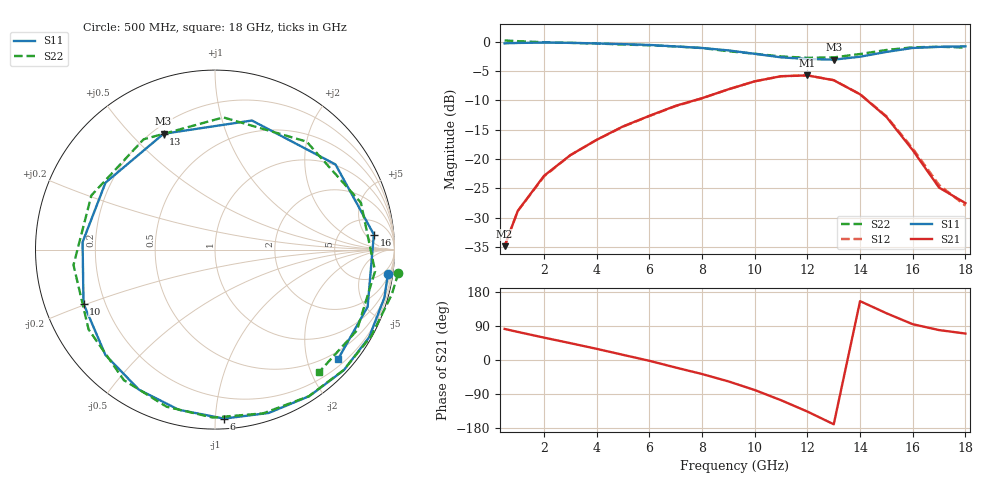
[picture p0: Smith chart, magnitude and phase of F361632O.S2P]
!ATF-36163
!VDS=2V VGS=-1.5V
! last updated 11-10-95
# ghz s ma r 50
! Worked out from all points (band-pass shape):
!   19 points, 500 MHz to 18 GHz, reference 50 ohm
!   highest |S21| = -5.71 dB at 12 GHz (marker M1); lowest = -34.9 dB at 500 MHz (marker M2)
!   |S21| within 3 dB of the highest: 8.588 GHz to 13.9 GHz (5.315 GHz wide, 47.3 % of centre)
!   lowest |S11| = -3.0 dB at 13 GHz (marker M3), VSWR 5.80, Z = 12.1 + j31.1 ohm
!   |S11| at or under -10 dB: nowhere
!   |S22| runs from -2.7 to 0.3 dB; largest |S21 - S12| = 0.0056
!   S11 on the Smith chart (normalised r, x): 500 MHz: 3, -14; 6 GHz: 0.06, -1.05; 10 GHz: 0.12, -0.19; 13 GHz: 0.24, +0.62; 16 GHz: 10, +8; 18 GHz: 0.33, -2.59
0.5  0.973 -8.1  0.018 81.9  0.018 80.9  1.03 -7.2
1  0.981 -15.9  0.036 74.1  0.036 73.4  1.016 -14.3
2  0.988 -29.7  0.072 59.0  0.071 58.8  0.995 -29.0
3  0.983 -43.1  0.108 44.4  0.108 44.5  0.982 -43.0
4  0.971 -57.2  0.146 29.4  0.146 29.5  0.97 -57.4
5  0.958 -71.8  0.19 13.6  0.189 13.7  0.951 -73.6
6  0.943 -86.9  0.234 -2.2  0.233 -2.3  0.936 -90.7
7  0.915 -102.7  0.285 -19.9  0.283 -20.0  0.916 -107.1
8  0.888 -118.5  0.331 -37.1  0.33 -37.2  0.887 -124.9
9  0.847 -136.1  0.394 -56.5  0.394 -56.5  0.833 -147.7
10  0.792 -157.7  0.461 -79.3  0.461 -79.3  0.793 -173.8
11  0.739 176.8  0.51 -106.2  0.509 -106.2  0.752 156.3
12  0.715 148.5  0.518 -136.1  0.518 -135.9  0.732 122.9
13  0.706 113.9  0.471 -169.6  0.472 -169.6  0.738 86.4
14  0.748 74.0  0.357 155.3  0.358 155.5  0.789 49.7
15  0.822 35.3  0.229 123.4  0.232 123.1  0.854 17.8
16  0.889 5.4  0.119 94.5  0.123 95.3  0.9 -7.7
17  0.908 -20.5  0.057 79.0  0.06 83.6  0.91 -29.7
18  0.918 -41.7  0.042 69.8  0.04 68.7  0.896 -49.8
